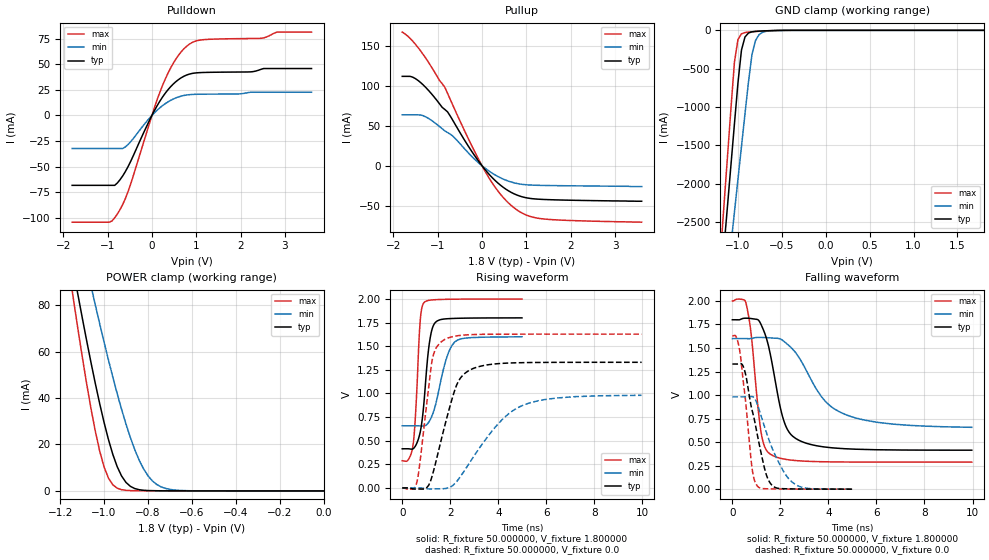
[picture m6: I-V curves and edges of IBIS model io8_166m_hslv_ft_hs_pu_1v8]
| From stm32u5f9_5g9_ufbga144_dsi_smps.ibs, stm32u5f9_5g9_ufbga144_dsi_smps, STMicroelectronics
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|   Model io8_166m_hslv_ft_hs_pu_1v8
[Model]  io8_166m_hslv_ft_hs_pu_1v8
Model_type I/O
Polarity   Non-Inverting
Enable   Active-Low
Vinl =   0.540000V
Vinh =   1.260000V
Vmeas =  0.900000V
Cref =   50.000000pF
Rref =   100.000000M
Vref =   0.0V
C_comp   3.358400pF   3.352800pF   3.400400pF
[Temperature Range]   25.000000   0.140000k   -40.000000
[Pullup Reference]   1.800000V   1.600000V   2.000000V
[Pulldown Reference]   0.0V   0.0V   0.0V
[POWER Clamp Reference]   1.800000V   1.600000V   2.000000V
[GND Clamp Reference]   0.0V   0.0V   0.0V
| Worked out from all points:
|   slope of the pulldown table from 0 to 0.27 V, typ, clamps not added: 13.6 ohm
|   slope of the pullup table from 0 to 0.27 V, typ, clamps not added: 15.9 ohm
|   GND clamp passes 1 mA (typ) near -0.51 V on its own axis
|   POWER clamp passes 1 mA (typ) near -0.86 V on its own axis
|   rising waveform, R_fixture 50.000000, V_fixture 1.800000: 20-80 % time 310ps typ, 545ps min, 202ps max; typ from 0.415 V to 1.8 V
|   rising waveform, R_fixture 50.000000, V_fixture 0.0: 20-80 % time 837ps typ, 1.81ns min, 451ps max; typ from 0 V to 1.33 V
|   falling waveform, R_fixture 50.000000, V_fixture 1.800000: 20-80 % time 689ps typ, 1.56ns min, 401ps max; typ from 1.8 V to 0.415 V
|   falling waveform, R_fixture 50.000000, V_fixture 0.0: 20-80 % time 637ps typ, 928ps min, 386ps max; typ from 1.33 V to 0 V
[Pulldown]
|Voltage   I(typ)   I(min)   I(max)
-1.8V     -68.38mA   -32.32mA   -104.4mA
-960mV    -68.38mA   -32.32mA   -104.4mA
-780mV    -66.08mA   -32.32mA   -96.43mA
-540mV    -50.22mA   -28.51mA   -74.66mA
0V        0A         0A         0A
240mV     18.04mA    9.6mA      29.42mA
480mV     30.68mA    16.02mA    50.95mA
780mV     39.48mA    19.99mA    67.56mA
1.14V     41.99mA    20.78mA    74.01mA
2.46V     45.1mA     22.69mA    75.45mA
2.82V     45.89mA    22.69mA    81.54mA
3.6V      45.89mA    22.69mA    81.54mA
[Pullup]
|Voltage   I(typ)   I(min)   I(max)
-1.8V     111.9mA    63.75mA    167.2mA
-1.56V    110.8mA    63.75mA    155.7mA
-1.26V    97.43mA    60.94mA    133.8mA
-840mV    70.48mA    43.76mA    98.29mA
-660mV    56.92mA    37.25mA    75.92mA
-300mV    23.77mA    15.64mA    32.82mA
120mV     -8.174mA   -5.123mA   -11.83mA
420mV     -24.43mA   -15.12mA   -35.87mA
720mV     -34.96mA   -21.23mA   -52.43mA
1.02V     -40.21mA   -23.8mA    -62.05mA
1.38V     -42.05mA   -24.52mA   -66.41mA
3.6V      -44.3mA    -26mA      -70.5mA
[GND_clamp]
|Voltage   I(typ)   I(min)   I(max)
-1.8V     -9.908A    -9.683A    -9.994A
-1.2V     -3.383A    -4.084A    -2.934A
-1.16V    -2.841A    -3.655A    -2.294A
-1.12V    -2.299A    -3.226A    -1.656A
-1.04V    -1.218A    -2.369A    -414.2mA
-1V       -684.7mA   -1.941A    -119.2mA
-960mV    -257.2mA   -1.514A    -45.66mA
-920mV    -87.03mA   -1.089A    -28.93mA
-840mV    -19.35mA   -312.8mA   -18.97mA
-800mV    -13.55mA   -132.4mA   -15.49mA
-720mV    -8.042mA   -25.67mA   -9.491mA
1.8V      0A         13.64nA    0A
[POWER_clamp]
|Voltage   I(typ)   I(min)   I(max)
-1.8V     470.9mA    433.7mA    554.6mA
-1.14V    95.28mA    122.7mA    82.88mA
-1.12V    85mA       114mA      70.34mA
-1.06V    55.55mA    88.43mA    35.73mA
-1.04V    46.38mA    80.17mA    25.83mA
-1V       29.54mA    64.14mA    10.37mA
-940mV    10.43mA    41.88mA    1.177mA
-900mV    3.66mA     28.79mA    250.5uA
-840mV    527.2uA    13.26mA    96.07uA
-800mV    154.2uA    6.55mA     88.1uA
-740mV    59.7uA     1.741mA    70.27uA
0V        0A         18.18nA    0A
[Ramp]
| variable   typ   min   max
dV/dt_r  0.79757/0.83546n   0.58660/1.80026n   0.97651/0.45001n
dV/dt_f  0.83120/0.68781n   0.56042/1.54050n   1.02743/0.40063n
R_load = 50.000000
[Rising Waveform]
R_fixture= 50.000000
V_fixture= 1.800000
V_fixture_min= 1.600000
V_fixture_max= 2.000000
|time   V(typ)   V(min)   V(max)
0s        414.5mV    657.5mV    287.8mV
450.5ps   414.9mV    657.7mV    454.4mV
560.6ps   449.5mV    657.7mV    812.5mV
740.7ps   582.5mV    656.8mV    1.744V
900.9ps   893.7mV    654.7mV    1.959V
1.141ns   1.553V     711.8mV    1.987V
1.401ns   1.757V     894.7mV    1.993V
1.842ns   1.79V      1.372V     1.996V
2.182ns   1.794V     1.545V     1.998V
4.985ns   1.8V       1.6V       1.999V
[Rising Waveform]
R_fixture= 50.000000
V_fixture= 0.0
V_fixture_min= 0.0
V_fixture_max= 0.0
|time   V(typ)   V(min)   V(max)
0s        382.6uV    497.2uV    514.2uV
620.6ps   -11.77mV   655.3uV    72.55mV
1.021ns   3.946mV    -8.813mV   895.5mV
1.241ns   123.4mV    -10.12mV   1.345V
1.702ns   589.3mV    -8.367mV   1.561V
2.322ns   1.121V     86.06mV    1.612V
3.003ns   1.269V     343.3mV    1.623V
4.164ns   1.318V     723.9mV    1.627V
5.085ns   1.326V     880.9mV    1.628V
9.97ns    1.33V      980.7mV    1.628V
[Falling Waveform]
R_fixture= 50.000000
V_fixture= 1.800000
V_fixture_min= 1.600000
V_fixture_max= 2.000000
|time   V(typ)   V(min)   V(max)
0s        1.8V       1.6V       1.999V
580.6ps   1.817V     1.6V       1.964V
780.8ps   1.813V     1.601V     1.653V
1.201ns   1.746V     1.613V     595.4mV
1.582ns   1.432V     1.607V     372.3mV
2.182ns   698.2mV    1.564V     318.9mV
2.823ns   513.4mV    1.381V     301mV
3.844ns   448.4mV    941.7mV    291.5mV
4.705ns   429.9mV    793.4mV    289.1mV
9.97ns    414.5mV    657.5mV    287.8mV
[Falling Waveform]
R_fixture= 50.000000
V_fixture= 0.0
V_fixture_min= 0.0
V_fixture_max= 0.0
|time   V(typ)   V(min)   V(max)
0s        1.33V      980.7mV    1.628V
150.2ps   1.33V      980.7mV    1.622V
290.3ps   1.332V     980.8mV    1.497V
500.5ps   1.269V     980.7mV    1.046V
820.8ps   838.6mV    984.6mV    221.4mV
1.031ns   588.9mV    907.4mV    36.58mV
1.341ns   219.3mV    661.8mV    5.556mV
1.542ns   78.49mV    511.5mV    3.882mV
2.442ns   3.382mV    85.7mV     1.369mV
4.985ns   382.6uV    497.2uV    514.2uV
